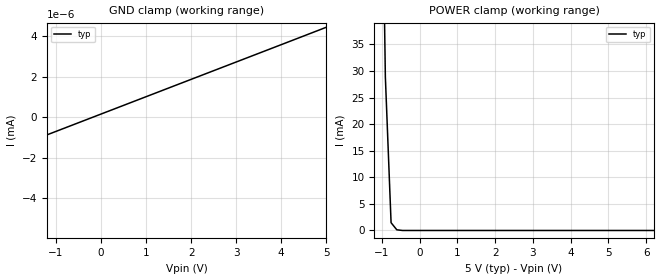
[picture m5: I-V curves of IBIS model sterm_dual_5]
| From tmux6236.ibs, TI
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| sterm_dual_5
[Model]   sterm_dual_5
Model_type   Terminator
|   typ   min   max
C_comp   2.533030e-11   NA   NA
[Voltage Range]   5   NA   NA
[Temperature Range]   27   NA   NA
[Power Clamp Reference]   5   NA   NA
[GND Clamp Reference]   0   NA   NA
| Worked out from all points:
|   GND clamp passes 1 mA (typ) near -5.68 V on its own axis
|   POWER clamp passes 1 mA (typ) near -0.70 V on its own axis
[GND Clamp]
|   Voltage   I(typ)   I(min)   I(max)
-10V      -6.86A     NA         NA
-5.303V   -22.09nA   NA         NA
-5.152V   -5.127nA   NA         NA
-5V       -4.133nA   NA         NA
5V        4.429nA    NA         NA
[POWER Clamp]
|   Voltage   I(typ)   I(min)   I(max)
-5V       7.062A     NA         NA
-1.061V   102.3mA    NA         NA
-909.1mV  28.93mA    NA         NA
-757.6mV  1.467mA    NA         NA
-606.1mV  126.8uA    NA         NA
-303mV    23.84nA    NA         NA
10V       -4.133nA   NA         NA
